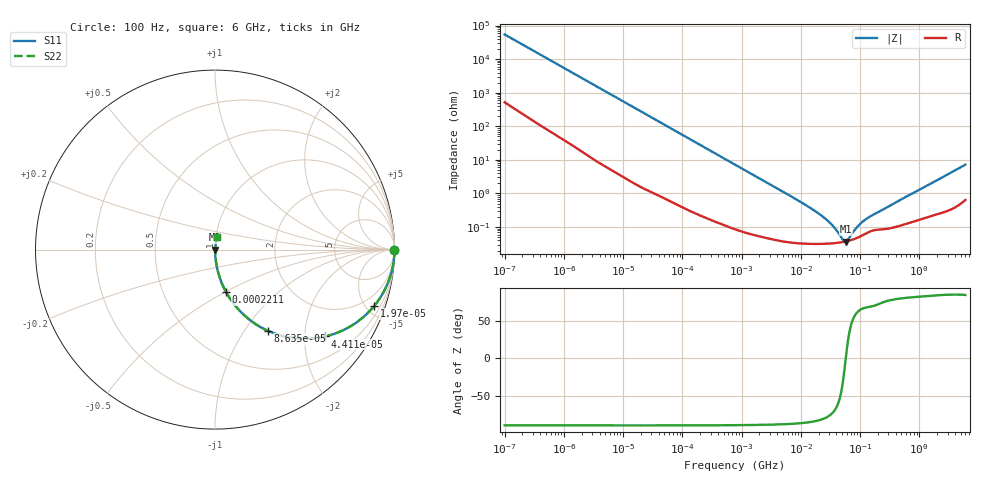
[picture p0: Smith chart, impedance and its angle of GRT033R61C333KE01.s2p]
!Murata Part Number: GRT033R61C333KE01
!These Parameters are Measured in Series Mode Connection
!Data Generated on Jun 19, 2026
!  o--ll--o
!Port1  Port2
!  o------o
!Operation Temp=25[degC], DC Bias Voltage=0[V]
!Freq. Start=100[Hz] Stop=6[GHz] 401[Steps]
# Hz S RI R 50
!Freq.(Hz) S11(Real) S11(Imag) S21(Real) S21(Imag) S12(Real) S12(Imag) S22(Real) S22(Imag)
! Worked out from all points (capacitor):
!   401 points, 100 Hz to 6 GHz, reference 50 ohm
!   read as one part in series: C = 29.2 nF near 109 Hz
!   lowest |Z| = 37.2 mohm at 56.99 MHz (marker M1)
!   series resonance near 57.4 MHz, so ESL is about 260 pH
!   S11 on the Smith chart (normalised r, x): 100 Hz: open; 19.7 kHz: 1.03, -5.64; 44.11 kHz: 1.02, -2.53; 86.35 kHz: 1.01, -1.30; 221.1 kHz: 1.00, -0.51; 6 GHz: 1.01, +0.14
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100  1 -0.00184  2.1e-05 0.00184  2.1e-05 0.00184  1 -0.00184
2008  0.9984 -0.0363  0.00155 0.0363  0.00155 0.0363  0.9984 -0.0363
7036  0.9835 -0.1247  0.0165 0.1247  0.0165 0.1247  0.9835 -0.1247
19704  0.8871 -0.3137  0.1129 0.3137  0.1129 0.3137  0.8871 -0.3137
28191  0.7945 -0.4011  0.2055 0.4011  0.2055 0.4011  0.7945 -0.4011
40335  0.6555 -0.4721  0.3445 0.4721  0.3445 0.4721  0.6555 -0.4721
44113  0.6144 -0.4836  0.3856 0.4836  0.3856 0.4836  0.6144 -0.4836
60352  0.4615 -0.4952  0.5385 0.4952  0.5385 0.4952  0.4615 -0.4952
86348  0.2967 -0.4534  0.7033 0.4534  0.7033 0.4534  0.2967 -0.4534
135116  0.1485 -0.352  0.8515 0.352  0.8515 0.352  0.1485 -0.352
221108  0.0622 -0.2376  0.9378 0.2376  0.9378 0.2376  0.0622 -0.2376
774597  0.00613 -0.0724  0.9939 0.0724  0.9939 0.0724  0.00613 -0.0724
1.555665e7  0.000327 -0.0034  0.9997 0.0034  0.9997 0.0034  0.000327 -0.0034
3.045065e7  0.000325 -0.00135  0.9997 0.00135  0.9997 0.00135  0.000325 -0.00135
3.80911e7  0.000334 -0.000837  0.9997 0.000837  0.9997 0.000837  0.000334 -0.000837
4.983056e7  0.000355 -0.00028  0.9996 0.00028  0.9996 0.00028  0.000355 -0.00028
5.699437e7  0.000372 -1.37e-05  0.9996 1.37e-05  0.9996 1.37e-05  0.000372 -1.37e-05
6.233367e7  0.000386 0.000163  0.9996 -0.000163  0.9996 -0.000163  0.000386 0.000163
8.918374e7  0.000478 0.00088  0.9995 -0.00088  0.9995 -0.00088  0.000478 0.00088
1.166697e8  0.000602 0.00144  0.9994 -0.00144  0.9994 -0.00144  0.000602 0.00144
3.124326e8  0.000929 0.00416  0.9991 -0.00416  0.9991 -0.00416  0.000929 0.00416
6e9  0.0114 0.0707  0.9886 -0.0707  0.9886 -0.0707  0.0114 0.0707
